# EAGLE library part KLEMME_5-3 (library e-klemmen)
Klemme 5 3
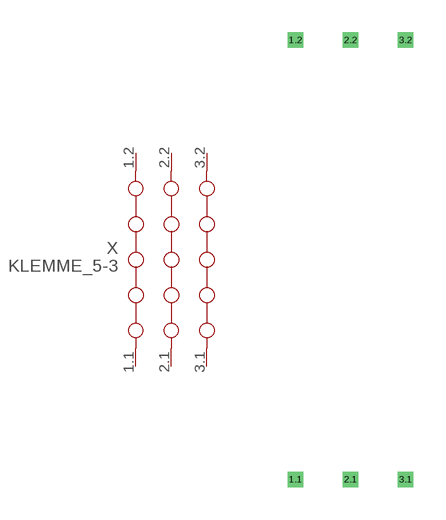
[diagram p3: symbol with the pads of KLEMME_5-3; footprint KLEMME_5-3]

Designator prefix X

## KLEMME_5-3  [KLEMME_5-3]
1.1  1.1  pas
1.2  1.2  pas
2.1  2.1  pas
2.2  2.2  pas
3.1  3.1  pas
3.2  3.2  pas

## Footprint KLEMME_5-3 (pad centres in mm)
Dummy
drill 0.2 pad 0.6 square: 1.1 -2.54,-10.16; 1.2 -2.54,10.16; 2.1 0,-10.16; 2.2 0,10.16; 3.1 2.54,-10.16; 3.2 2.54,10.16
